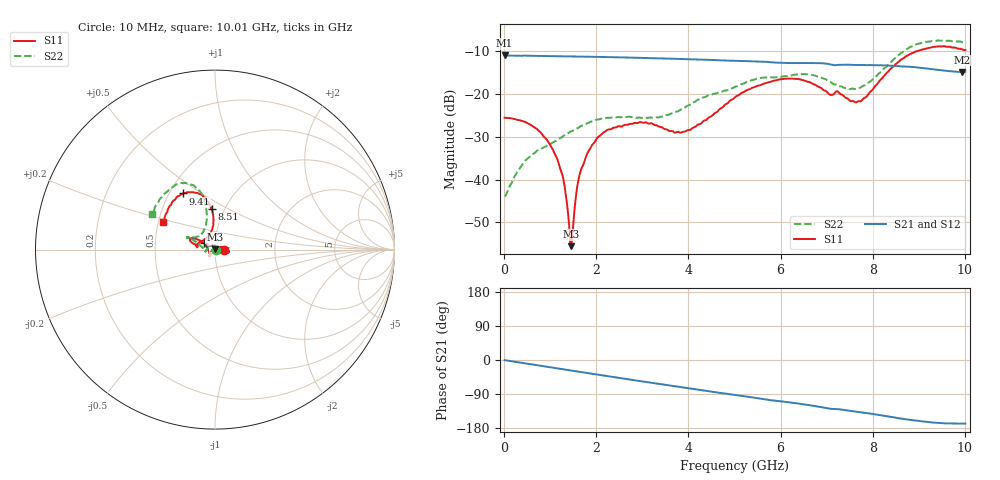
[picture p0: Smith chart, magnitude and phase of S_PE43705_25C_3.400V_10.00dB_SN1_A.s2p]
! Device ID: PE43705
! Serial: 1
! Insertion: A
! Impedance: 50 ohm
! Temp: 25C
! VDD: 3.400V
! Attenuation Step: 10.00dB
#  Hz  S  RI  R  50
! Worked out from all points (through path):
!   401 points, 10 MHz to 10.01 GHz, reference 50 ohm
!   highest |S21| = -10.98 dB at 10 MHz (marker M1); lowest = -14.8 dB at 9.935 GHz (marker M2)
!   group delay of S21, straight-line fit = 48.4 ps
!   lowest |S11| = -55.6 dB at 1.46 GHz (marker M3), VSWR 1.00, Z = 49.8 + j0.0626 ohm
!   |S11| at or under -10 dB: start of sweep to 8.946 GHz
!   |S22| runs from -44.0 to -7.5 dB; largest |S21 - S12| = 0.0022
!   S11 on the Smith chart (normalised r, x): 10 MHz: 1.11, +0.00; 4.76 GHz: 0.88, +0.06; 8.51 GHz: 0.87, +0.41; 9.41 GHz: 0.59, +0.42; 10.01 GHz: 0.53, +0.18
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1e7  0.0528 4.14e-05  0.2824 -0.0013  0.2826 -0.00119  0.00633 0.000365
4.6e8  0.0453 0.0124  0.2769 -0.0442  0.277 -0.0437  0.00253 0.0165
1.01e9  0.0211 0.013  0.2616 -0.093  0.2616 -0.0927  -0.0165 0.0201
1.26e9  0.00898 0.00718  0.252 -0.1132  0.2522 -0.113  -0.0266 0.0166
1.41e9  0.000964 0.00277  0.2455 -0.1251  0.2456 -0.125  -0.0328 0.0136
1.46e9  -0.00154 0.000628  0.2431 -0.129  0.2432 -0.1288  -0.0347 0.012
1.585e9  -0.00754 -0.00323  0.2369 -0.1384  0.2371 -0.1383  -0.0387 0.00884
1.685e9  -0.0114 -0.00768  0.2319 -0.1458  0.232 -0.1456  -0.0422 0.00598
1.885e9  -0.019 -0.0147  0.221 -0.1598  0.2211 -0.1596  -0.0476 0.000604
2.21e9  -0.0252 -0.0271  0.2014 -0.1808  0.2015 -0.1807  -0.0518 -0.00761
3.36e9  -0.0279 -0.0309  0.1185 -0.2327  0.1187 -0.2325  -0.0532 -0.00505
3.885e9  -0.0351 -0.00834  0.0772 -0.2445  0.0774 -0.2443  -0.0667 0.00907
4.76e9  -0.062 0.0359  0.00884 -0.2469  0.00936 -0.247  -0.1006 0.0405
5.01e9  -0.078 0.0481  -0.00974 -0.2445  -0.00947 -0.2445  -0.1119 0.0473
5.985e9  -0.1344 0.063  -0.0751 -0.2195  -0.0739 -0.2196  -0.1432 0.0678
6.685e9  -0.1272 0.0374  -0.1165 -0.1983  -0.1165 -0.1984  -0.1512 0.0683
7.685e9  -0.0454 0.0688  -0.1599 -0.1491  -0.1598 -0.1494  -0.0689 0.0954
8.36e9  -0.00945 0.19  -0.1848 -0.1099  -0.1844 -0.1102  -0.0483 0.2229
8.51e9  -0.0188 0.2251  -0.1882 -0.0974  -0.1872 -0.0988  -0.0565 0.2627
9.41e9  -0.1784 0.3128  -0.186 -0.0459  -0.1857 -0.046  -0.2204 0.361
9.935e9  -0.2804 0.1811  -0.1771 -0.0383  -0.1777 -0.0386  -0.3373 0.2249
1.001e10  -0.2894 0.1532  -0.1778 -0.0386  -0.1785 -0.0393  -0.3511 0.1969
